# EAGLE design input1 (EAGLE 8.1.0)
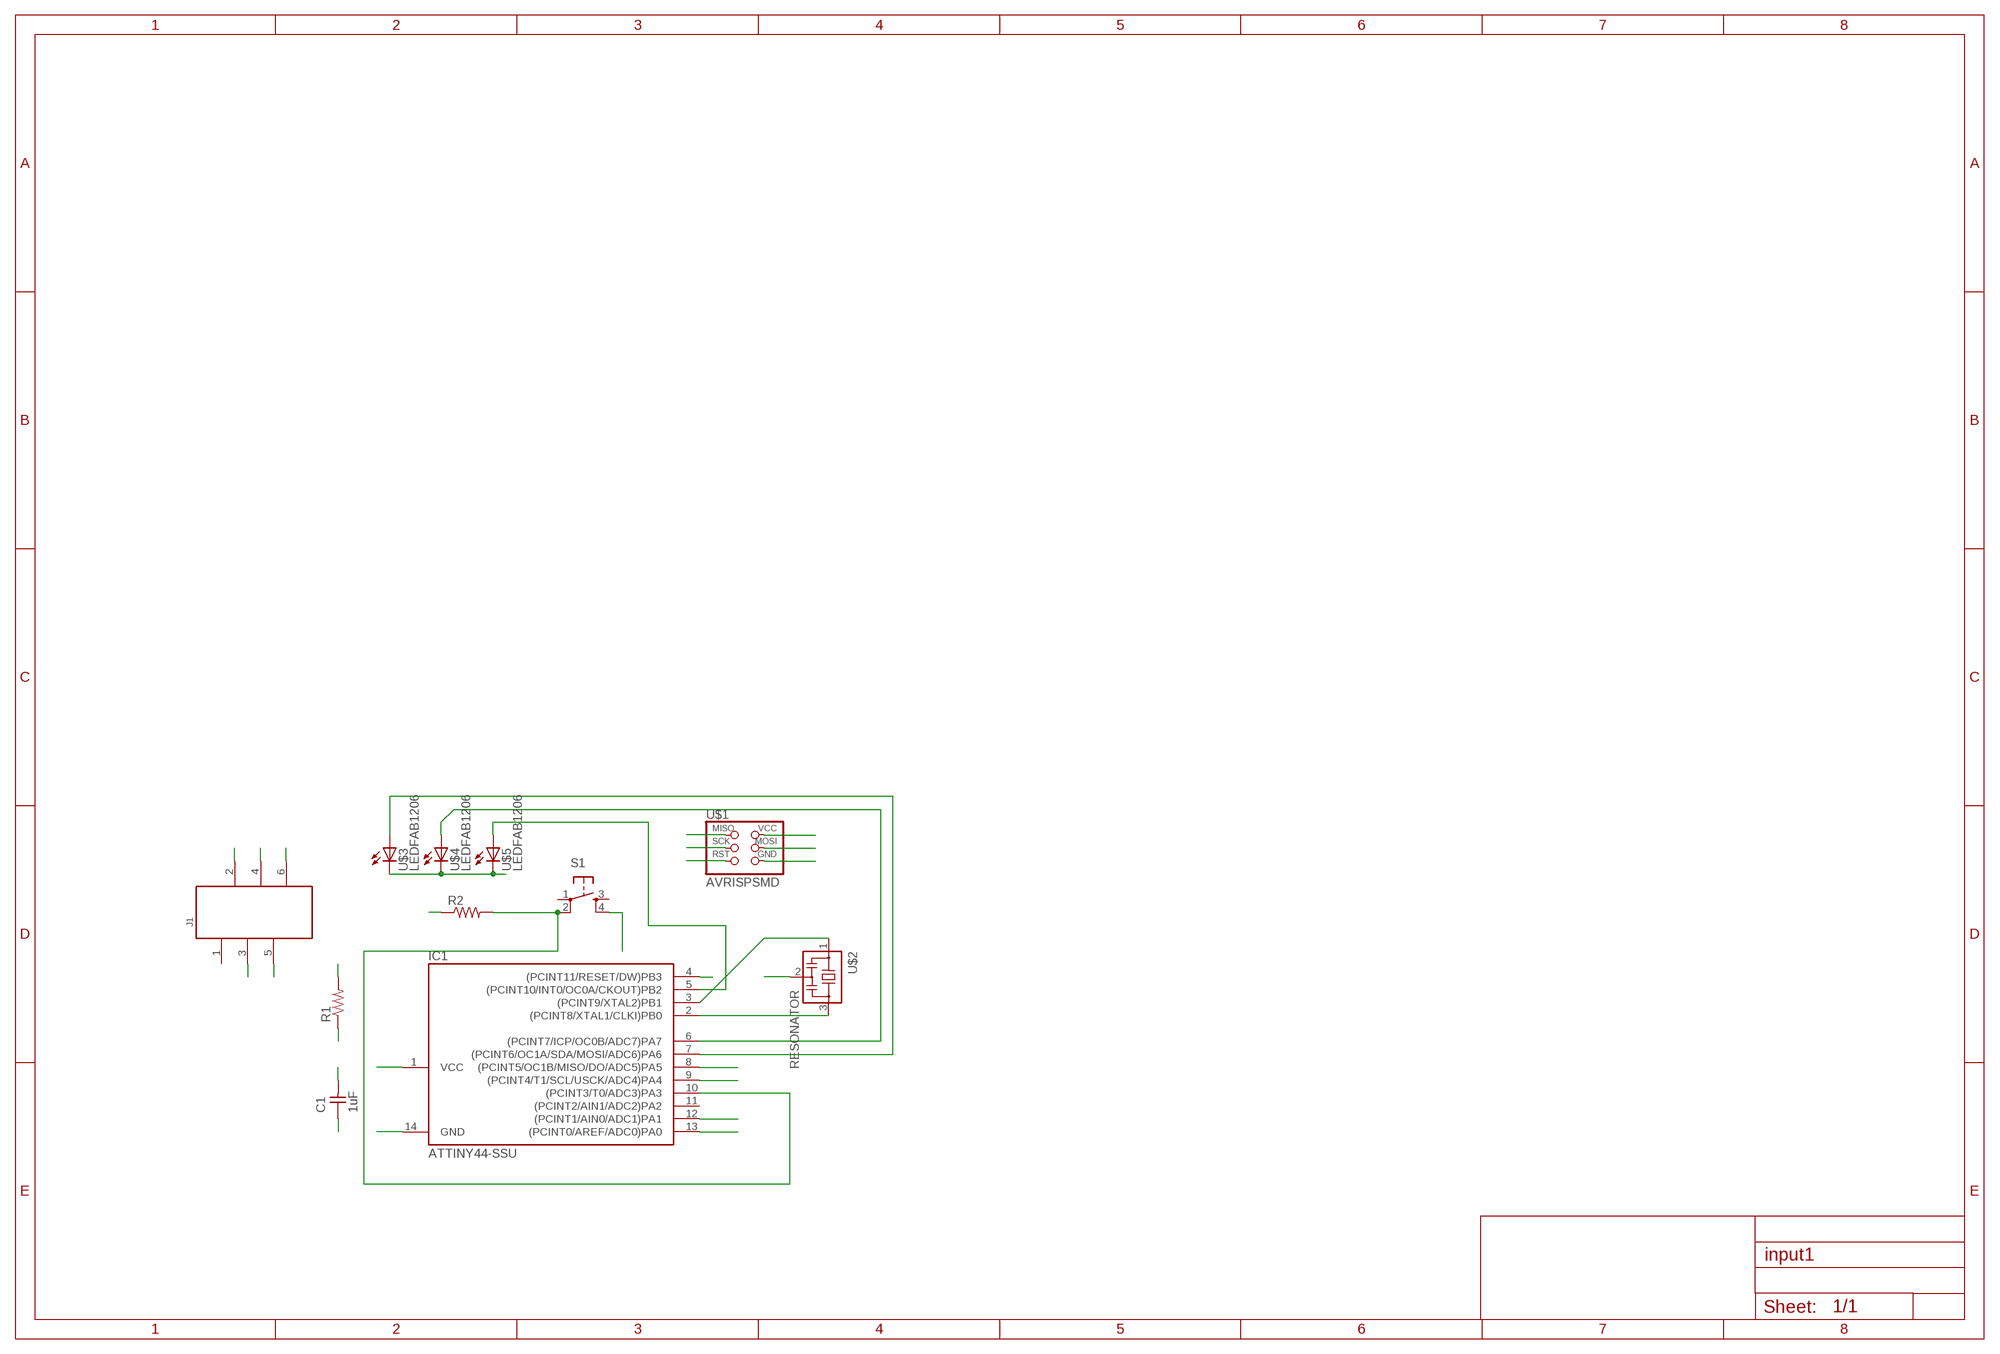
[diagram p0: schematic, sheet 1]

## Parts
C1  1uF  CAP-UNPOLARIZEDFAB  [C1206FAB]
IC1  ATTINY44-SSU  [SOIC14]
J1  61000618221  [61000618221]
R1  RES-US1206FAB  [R1206FAB]
R2  RES-US1206FAB  [R1206FAB]
S1  6MM_SWITCH6MM_SWITCH  [6MM_SWITCH]
U$1  AVRISPSMD  [2X03SMD]
U$2  RESONATOR  [EFOBM]
U$3  LEDFAB1206  [LED1206FAB]
U$4  LEDFAB1206  [LED1206FAB]
U$5  LEDFAB1206  [LED1206FAB]

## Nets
GND: C1.1 IC1.14(GND) J1.6 R2.1 U$1.6(GND) U$2.2 U$3.2(C) U$4.2(C) U$5.2(C)
MISO: IC1.8((PCINT5/OC1B/MISO/DO/ADC5)PA5) U$1.1(MISO)
MOSI: IC1.7((PCINT6/OC1A/SDA/MOSI/ADC6)PA6) U$1.4(MOSI) U$3.1(A)
N$2: IC1.3((PCINT9/XTAL2)PB1) U$2.1
N$3: IC1.2((PCINT8/XTAL1/CLKI)PB0) U$2.3
N$4: IC1.6((PCINT7/ICP/OC0B/ADC7)PA7) U$4.1(A)
N$5: IC1.5((PCINT10/INT0/OC0A/CKOUT)PB2) U$5.1(A)
N$6: IC1.10((PCINT3/T0/ADC3)PA3) R2.2 S1.2(P1)
N$7: J1.5
RST: IC1.4((PCINT11/RESET/DW)PB3) R1.1 U$1.5(RST)
RX: IC1.12((PCINT1/AIN0/ADC1)PA1) J1.2
SCK: IC1.9((PCINT4/T1/SCL/USCK/ADC4)PA4) U$1.3(SCK)
TX: IC1.13((PCINT0/AREF/ADC0)PA0) J1.3
VCC: C1.2 IC1.1(VCC) J1.4 R1.2 S1.4(S1) U$1.2(VCC)
Unconnected: IC1.11((PCINT2/AIN1/ADC2)PA2) J1.1 S1.1(P) S1.3(S)

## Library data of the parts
C1 = fab:CAP-UNPOLARIZED
IC1 = fab:ATTINY44
J1 = EAGLE-BOARD-TO-BOARD_CONNECTORS-rev16c:61000618221: WR-PHD 2.54mm SMT Pin Header, 6 Pins =>Code : Con_BTB_PHD_2.54_1_SMT_61000618221 Details see: http://katalog.we-online.de/en/em/610_0xx_182_21 Created 2014-05-29, Karrer Zheng 2014 (C) Würth Elektronik
R1 R2 = fab:RES-US: Resistor (US Symbol)
S1 = fab:6MM_SWITCH: OMRON SWITCH
U$1 = fab:AVRISP
U$2 = fab:RESONATOR
U$3-U$5 = fab:LED: LED

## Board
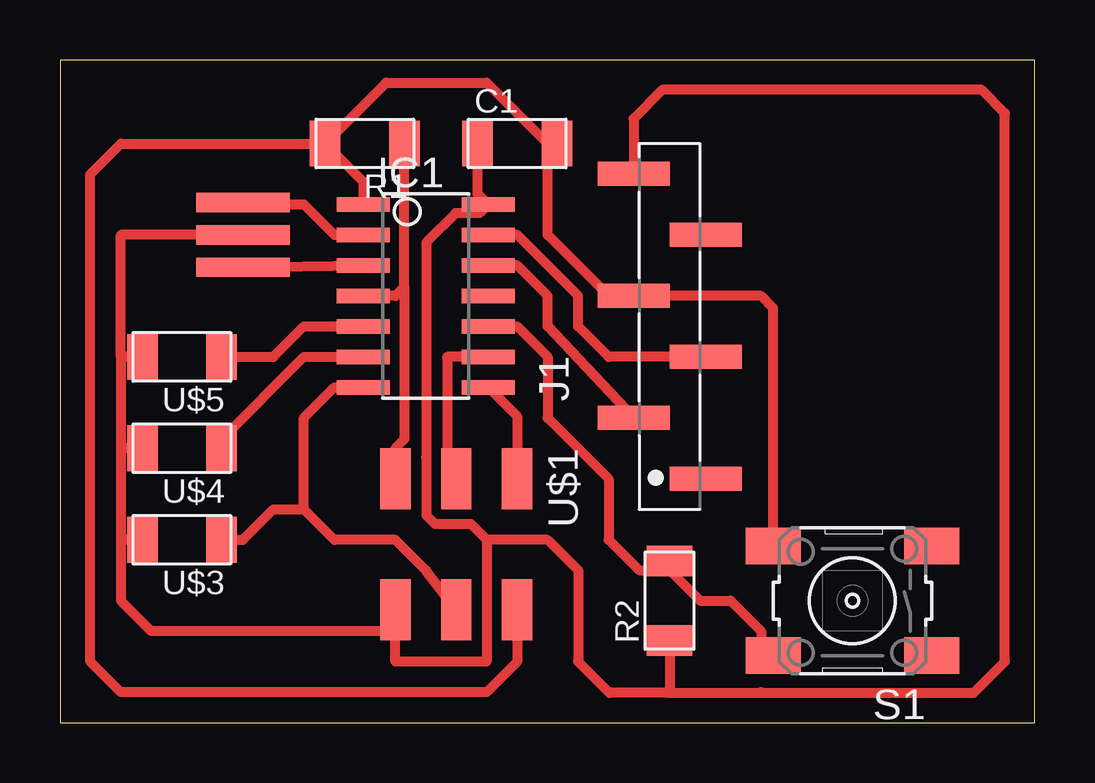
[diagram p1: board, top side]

Size 40.62 x 27.61 mm. Coordinates in mm from the lower left corner, seen from the top.
Outline: 0,0 40.62,0 40.62,27.61 0,27.61 0,0
Copper layers (1*16): Top 0.035mm / dielectric 1.5mm / Bottom 0.035mm
Design rules "default *": minimum track width 10mil, minimum drill 24mil, track to track 16mil, track to pad 16mil, pad to pad 16mil, via to via 16mil, smd to smd 16mil, copper to edge 40mil, drill to drill 8mil, minimum pad ring 10mil, minimum via ring 8mil, stop-mask expansion 4mil, vias tented up to drill 0mil, thermal gap 10mil

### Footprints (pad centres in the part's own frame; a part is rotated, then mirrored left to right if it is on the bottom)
C1206FAB = smd 1.27 x 1.905: 1 -1.651,0; 2 1.651,0
SOIC14 = smd 0.61 x 2.21: 1 -3.81,-2.603; 2 -2.54,-2.603; 3 -1.27,-2.603; 4 0,-2.603; 5 1.27,-2.603; 6 2.54,-2.603; 7 3.81,-2.603; 8 3.81,2.603; 9 2.54,2.603; 10 1.27,2.603; 11 0,2.603; 12 -1.27,2.603; 13 -2.54,2.603; 14 -3.81,2.603
61000618221 = smd 1 x 3: 1 -6.35,-1.5; 2 -3.81,1.5; 3 -1.27,-1.5; 4 1.27,1.5; 5 3.81,-1.5; 6 6.35,1.5
R1206FAB = smd 1.27 x 1.905: 1 -1.651,0; 2 1.651,0
6MM_SWITCH = smd 2.286 x 1.524: 1 -3.302,2.286; 2 3.302,2.286; 3 -3.302,-2.286; 4 3.302,-2.286
2X03SMD = smd 2.54 x 1.27: 1 -2.54,2.54; 2 2.92,2.54; 3 -2.54,0; 4 2.92,0; 5 -2.54,-2.54; 6 2.92,-2.54
EFOBM = smd 0.8 x 3.9: 1 -1.35,0; 2 0,0; 3 1.35,0
LED1206FAB = smd 1.27 x 1.905: 1 -1.651,0; 2 1.651,0

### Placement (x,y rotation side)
C1  19.05,24.13 0 top
IC1  15.24,17.78 270 top
J1  25.4,16.51 90 top
R1  12.7,24.13 180 top
R2  25.4,5.08 90 top
S1  33.02,5.08 180 top
U$1  16.51,7.62 270 top
U$2  7.62,20.32 90 top
U$3  5.08,7.62 180 top
U$4  5.08,11.43 180 top
U$5  5.08,15.24 180 top

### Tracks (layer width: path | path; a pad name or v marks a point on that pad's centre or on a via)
GND
  Top 0.406: C1.1 17.4,22.03 IC1.14 17.49,21.23 16.49,21.23 15.26,20.01 15.26,11.08 15.25,11.04 15.26,11 15.26,8.64 15.62,8.28 17.12,8.28 17.78,7.62 | U$2.2 2.54,20.32 2.54,15.24 | 2.54,11.43 2.54,7.62 | 2.54,15.24 2.54,11.43 | 2.54,7.62 2.54,5.08 3.81,3.81 13.97,3.81 | 13.97,3.81 U$1.6 | 17.78,7.62 17.78,2.54 13.97,2.54 13.97,3.81 | U$3.2 2.54,7.62 | U$4.2 2.54,11.43 | U$5.2 2.54,15.24 | J1.6 23.9,25.17 25.12,26.39 38.38,26.39 39.37,25.4 39.37,2.54 38.07,1.24 29.24,1.24 | 29.21,1.27 29.24,1.24 | 25.4,1.24 29.24,1.24 | 25.4,1.24 22.89,1.24 21.59,2.54 21.59,6.35 20.32,7.62 17.78,7.62 | R2.1 25.4,1.24
MISO
  Top 0.406: IC1.8 19.05,12.76 U$1.1
MOSI
  Top 0.406: U$1.4 15.24,6.35 13.97,7.62 11.43,7.62 10.16,8.89 | IC1.7 11.43,13.97 10.16,12.7 10.16,8.89 | U$3.1 7.62,7.62 8.89,8.89 10.16,8.89
N$2
  Top 0.406: U$2.1 IC1.3
N$3
  Top 0.406: U$2.3 6.35,21.59 10.16,21.59 11.43,20.32 IC1.2
N$4
  Top 0.406: U$4.1 6.73,11.81 10.16,15.24 IC1.6
N$5
  Top 0.406: U$5.1 8.89,15.24 10.16,16.51 IC1.5
N$6
  Top 0.406: IC1.10 19.05,16.51 20.32,15.24 20.32,12.7 22.86,10.16 22.86,7.62 24.13,6.35 25.02,6.35 R2.2 25.4,6.35 26.67,5.08 27.94,5.08 29.21,3.81 29.21,3.3 S1.2
RST
  Top 0.406: 14.35,18.16 13.97,17.78 IC1.4 | 14.35,18.16 R1.1 | 14.35,18.16 14.35,11.81 13.97,11.43 U$1.5
RX
  Top 0.406: J1.2 20.32,16.51 20.32,17.78 19.05,19.05 IC1.12
SCK
  Top 0.406: IC1.9 16.13,15.24 16.13,11.05 U$1.3
TX
  Top 0.406: J1.3 22.86,15.24 21.59,16.51 21.59,17.78 19.05,20.32 IC1.13
VCC
  Top 0.406: R1.2 12.64,22.54 IC1.1 | R1.2 13.59,26.67 17.78,26.67 20.32,24.13 C1.2 20.32,23.75 20.32,20.32 22.86,17.78 J1.4 29.21,17.78 29.72,17.27 S1.4 | U$1.2 19.05,2.54 17.78,1.27 2.54,1.27 1.27,2.54 1.27,22.86 2.54,24.13 R1.2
